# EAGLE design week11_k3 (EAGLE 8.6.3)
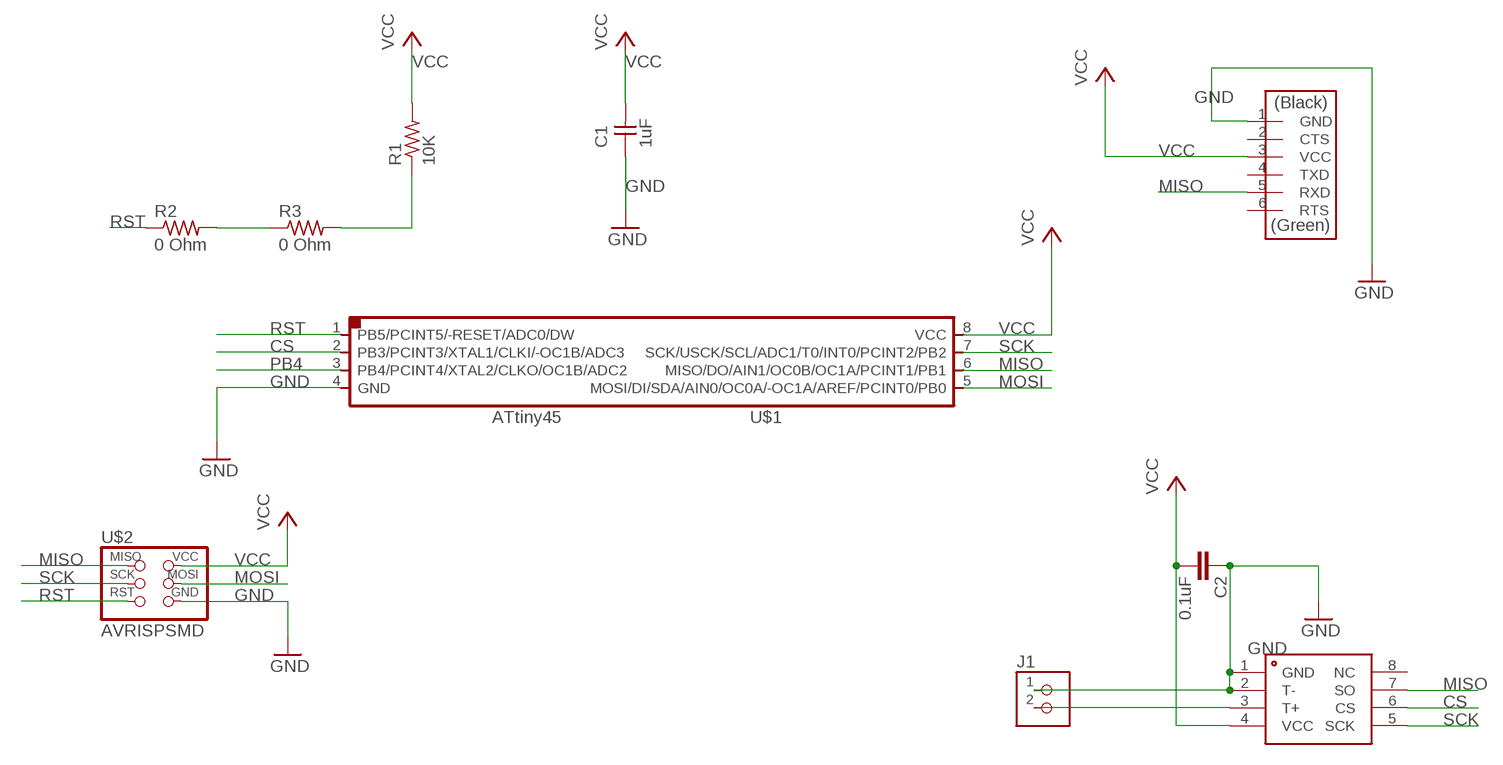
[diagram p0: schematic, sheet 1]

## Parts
C1  1uF  CAP-UNPOLARIZEDFAB  [C1206FAB]
C2  0.1uF  C-EUC0805K  [C0805K]
J1  TERM-1X02-ADAFRUIT  [3.5MMTERM]
MAX6675  MAX6675  [SO08]
R1  10K  RES-US1206FAB  [R1206FAB]
R2  0 Ohm  RES-US1206FAB  [R1206FAB]
R3  0 Ohm  RES-US1206FAB  [R1206FAB]
U$1  ATTINY45SI  [SOIC8]
U$2  AVRISPSMD  [2X03SMD]
U$3  FTDI-SMD-HEADER  [1X06SMD]

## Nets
CS: MAX6675.6(CS) U$1.2(PB3/PCINT3/XTAL1/CLKI/-OC1B/ADC3)
GND: C1.1 C2.1 J1.1 MAX6675.1(GND) MAX6675.2(T-) U$1.4(GND) U$2.6(GND) U$3.1(GND)
MISO: MAX6675.7(SO) U$1.6(MISO/DO/AIN1/OC0B/OC1A/PCINT1/PB1) U$2.1(MISO) U$3.5(RXD)
MOSI: U$1.5(MOSI/DI/SDA/AIN0/OC0A/-OC1A/AREF/PCINT0/PB0) U$2.4(MOSI)
N$1: J1.2 MAX6675.3(T+)
PB4: U$1.3(PB4/PCINT4/XTAL2/CLKO/OC1B/ADC2)
RST: R1.1 R2.1 R2.2 R3.1 R3.2 U$1.1(PB5/PCINT5/-RESET/ADC0/DW) U$2.5(RST)
SCK: MAX6675.5(SCK) U$1.7(SCK/USCK/SCL/ADC1/T0/INT0/PCINT2/PB2) U$2.3(SCK)
VCC: C1.2 C2.2 MAX6675.4(VCC) R1.2 U$1.8(VCC) U$2.2(VCC) U$3.3(VCC)
Unconnected: MAX6675.8(NC) U$3.2(CTS) U$3.4(TXD) U$3.6(RTS)

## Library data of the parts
C1 = fab:CAP-UNPOLARIZED
C2 = resistor:C-EU: CAPACITOR, European symbol
J1 = fab:TERM-1X02: 3.5mm terminal block, 2 positions ED555-2DS as found in the fablab inventory.
MAX6675 = maxim:MAX6675
R1-R3 = fab:RES-US: Resistor (US Symbol)
U$1 = fab:ATTINY45
U$2 = fab:AVRISP
U$3 = fab:FTDI-SMD-HEADER

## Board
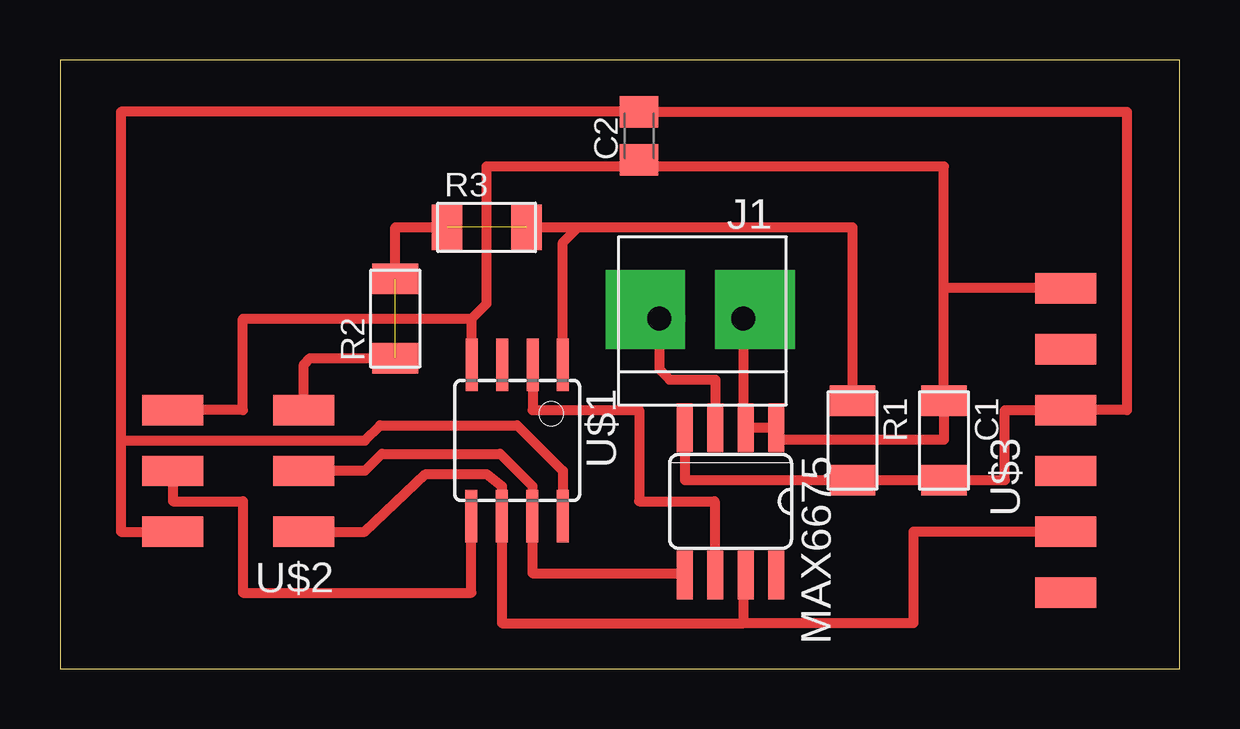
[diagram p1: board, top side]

Size 46.66 x 25.39 mm. Coordinates in mm from the lower left corner, seen from the top.
Outline: 0,0 46.66,0 46.66,25.39 0,25.39 0,0
Copper layers (1*16): Top 0.035mm / dielectric 1.5mm / Bottom 0.035mm
Design rules "default *": minimum track width 6mil, minimum drill 0.35mm, track to track 0.04mm, track to pad 0.04mm, pad to pad 0.04mm, via to via 0.04mm, smd to smd 0.04mm, copper to edge 40mil, drill to drill 6mil, minimum pad ring 10mil, minimum via ring 8mil, stop-mask expansion 4mil, vias tented up to drill 0mil, thermal gap 10mil

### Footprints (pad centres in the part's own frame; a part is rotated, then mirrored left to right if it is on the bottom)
C1206FAB = smd 1.27 x 1.905: 1 -1.651,0; 2 1.651,0
C0805K = smd 1.3 x 1.6: 1 -1,0; 2 1,0
3.5MMTERM = drill 1 pad 2.184: 1 1.8,0; 2 -1.7,0
SO08 = smd 0.66 x 2.032: 1 -1.905,-3.073; 2 -0.635,-3.073; 3 0.635,-3.073; 4 1.905,-3.073; 5 1.905,3.073; 6 0.635,3.073; 7 -0.635,3.073; 8 -1.905,3.073
R1206FAB = smd 1.27 x 1.905: 1 -1.651,0; 2 1.651,0
SOIC8 = smd 0.5 x 2.2: 1 -1.905,-3.154; 2 -0.645,-3.154; 3 0.625,-3.154; 4 1.895,-3.154; 5 1.905,3.154; 6 0.635,3.154; 7 -0.635,3.154; 8 -1.905,3.154
2X03SMD = smd 2.54 x 1.27: 1 -2.54,2.54; 2 2.92,2.54; 3 -2.54,0; 4 2.92,0; 5 -2.54,-2.54; 6 2.92,-2.54
1X06SMD = smd 2.54 x 1.27: 1 0,6.35; 2 0,3.81; 3 0,1.27; 4 0,-1.27; 5 0,-3.81; 6 0,-6.35

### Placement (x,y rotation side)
C1  36.83,9.53 270 top
C2  24.13,22.23 90 top
J1  26.67,14.61 0 top
MAX6675  27.94,6.99 180 top
R1  33.02,9.53 270 top
R2  13.97,14.61 90 top
R3  17.78,18.41 0 top
U$1  19.05,9.53 180 top
U$2  7.62,8.26 180 top
U$3  41.91,9.53 0 top

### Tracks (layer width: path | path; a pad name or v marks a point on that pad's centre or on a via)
CS
  Top 0.152: 27.28,4.6 27.28,4.45 27.28,3.99 MAX6675.6 | 19.81,12.06 19.81,12.68 U$1.2
  Top 0.406: U$1.2 19.7,10.79 24.13,10.79 24.13,6.99 27.28,6.99 27.28,4.45
GND
  Top 0.152: 28.65,10.08 MAX6675.2 | 29.72,10.08 MAX6675.1 29.87,10.08 | 37.34,11.3 36.88,11.3 C1.1 36.74,11.15 36.73,11.15 | 4.72,10.85 U$2.6 | 17.07,12.68 U$1.4
  Top 0.406: 36.74,11.15 36.83,11.15 36.83,9.55 29.72,9.55 29.72,10.08 | C2.1 24.13,20.95 | 24.13,20.95 36.83,20.95 36.83,15.88 | C1.1 36.83,15.88 | U$1.4 17.16,14.61 | 4.72,10.85 4.72,10.79 7.62,10.79 7.62,14.61 17.16,14.61 | MAX6675.1 MAX6675.2 28.47,10.16 J1.1 | 17.16,14.61 17.78,15.23 17.78,20.95 24.13,20.95 | U$3.1 36.83,15.88
MISO
  Top 0.152: 28.5,3.38 28.5,3.83 MAX6675.7 | 18.44,5.82 18.44,6.27 U$1.6 | 10.21,5.82 U$2.1
  Top 0.406: U$3.5 35.56,5.71 35.56,1.91 28.5,1.91 | 28.5,1.91 28.5,3.38 | 28.5,1.91 18.41,1.91 U$1.6 18.41,7.62 17.78,8.13 15.24,8.13 12.7,5.71 U$2.1
MOSI
  Top 0.406: U$2.4 4.7,6.99 7.62,6.99 7.62,3.17 17.14,3.17 U$1.5
N$1
  Top 0.406: J1.2 24.97,12.49 25.4,12.06 27.3,12.06 MAX6675.3
N$2  (via drill 0 pad 3.3)
  other vias: 24.38,14.99
N$3  (via drill 0 pad 3.3)
  other vias: 28.96,14.99
RST  (2 unrouted)
  Top 0.152: 21.03,12.68 U$1.1
  Top 0.406: R2.2 13.97,18.41 R3.1 | R3.2 21.59,18.41 | 21.59,18.41 33.02,18.41 R1.1 | U$1.1 20.95,17.78 21.59,18.41 | U$2.5 10.16,12.7 10.41,12.95 R2.1
SCK
  Top 0.152: 19.81,5.82 19.81,6.27 U$1.7 | 25.91,3.99 MAX6675.5
  Top 0.406: U$2.3 12.7,8.26 13.41,8.97 18.34,8.97 19.68,7.62 U$1.7 19.68,3.99 25.91,3.99
VCC
  Top 0.152: 33.07,7.95 R1.2 32.92,7.95 | 36.73,7.95 C1.2 36.88,7.95 | 26.06,9.63 26.06,9.93 MAX6675.4 | 41.91,10.85 U$3.3 41.91,10.69
  Top 0.406: MAX6675.4 26.04,7.87 R1.2 36.88,7.87 36.88,7.95 | C1.2 39.37,7.87 39.37,10.79 U$3.3 44.45,10.79 44.45,23.23 C2.2 2.54,23.23 2.54,9.53 | 2.54,9.53 2.54,5.71 U$2.2 | 2.54,9.53 12.7,9.53 13.34,10.16 19.05,10.16 20.95,8.26 U$1.8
